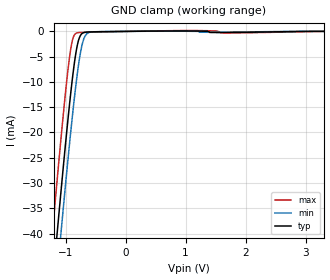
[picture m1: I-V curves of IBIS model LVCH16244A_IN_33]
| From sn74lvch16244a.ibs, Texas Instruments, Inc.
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[Model]   LVCH16244A_IN_33
Model_type  Input
Vinl=0.8
Vinh=2.0
| variable   typ   min   max
C_comp   3.15pF   2.47pF   4.35pF
[Temperature Range]   40   100   -40
| Ambient temperature   25   85   -40
[Voltage range]   3.3   3   3.6
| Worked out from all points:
|   GND clamp passes 1 mA (typ) near -0.76 V on its own axis
[GND Clamp]
| LVCH16244A_IN_33
|   Voltage   I(typ)   I(min)   I(max)
-5V       -584.8mA   -591.6mA   -576.5mA
-1.215V   -49.86mA   -58.06mA   -39.36mA
-1.14V    -39.97mA   -48.18mA   -29.44mA
-1.08V    -32.21mA   -40.4mA    -21.73mA
-985mV    -20.41mA   -28.44mA   -10.34mA
-920mV    -12.94mA   -20.66mA   -3.999mA
-875mV    -8.304mA   -15.57mA   -1.329mA
-820mV    -3.745mA   -9.886mA   -353.2uA
-770mV    -1.281mA   -5.549mA   -236.6uA
-715mV    -345.6uA   -2.223mA   -207.4uA
-590mV    -112.5uA   -155.9uA   -164.6uA
3.3V      9.604pA    40.35nA    -142.3nA
